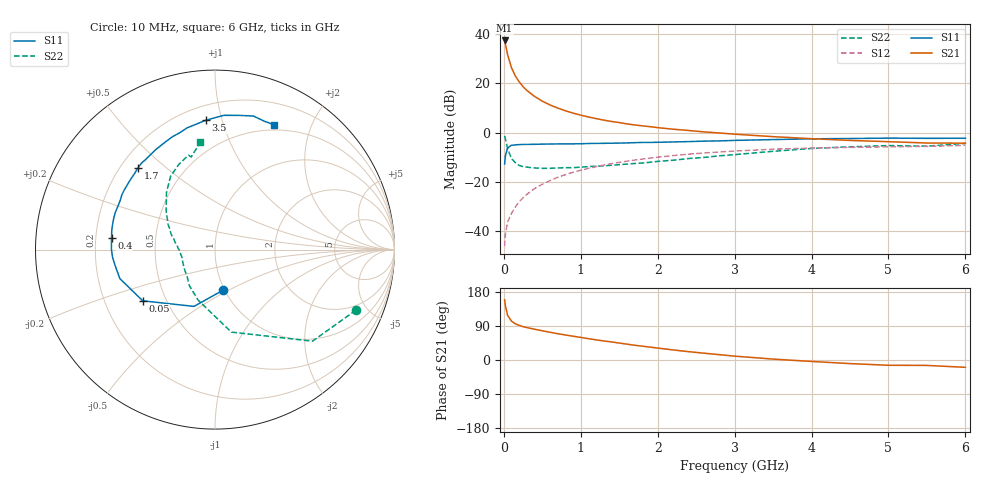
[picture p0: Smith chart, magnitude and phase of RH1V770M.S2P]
! SIEMENS Small Signal Semiconductors
! BFR106
! Si NPN RF Bipolar Junction Transistor in SOT23
! VCE = 1.75 V  IC = 70 mA
! Common Emitter S-Parameters:  August  1996
# GHz  S  MA  R  50
!  f  S11  S21  S12  S22
! GHz  MAG  ANG  MAG  ANG  MAG  ANG  MAG  ANG
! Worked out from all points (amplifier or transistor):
!   36 points, 10 MHz to 6 GHz, reference 50 ohm
!   highest |S21| = 37.4 dB at 10 MHz (marker M1)
!   |S21| within 3 dB of that: start of sweep to 30.49 MHz
!   unconditionally stable (mu >= 1): 180.2 MHz to 2.981 GHz; 4.611 GHz to end of sweep
!   at 250 MHz: K = 1.05, MAG = 21.1 dB, |S12| = -26.4 dB
!   at 1.4 GHz: K = 1.07, MAG = 6.9 dB, |S12| = -12.6 dB
!   at 6 GHz: K = 1.01, MAG = -0.3 dB, |S12| = -5.1 dB
!   S11 on the Smith chart (normalised r, x): 10 MHz: 0.98, -0.47; 50 MHz: 0.37, -0.28; 400 MHz: 0.27, +0.05; 1.7 GHz: 0.27, +0.41; 3.5 GHz: 0.29, +0.89; 6 GHz: 0.44, +1.49
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0.01  0.2316 -79.5  73.8 158.8  0.005 77.5  0.8551 -23.2
0.02  0.3375 -110.3  62.68 142.9  0.0089 66.5  0.7452 -43.2
0.05  0.4936 -144.7  37.23 117.4  0.0155 59.2  0.4686 -78.8
0.1  0.5543 -163.1  20.63 102.4  0.0232 63.7  0.2972 -108.3
0.15  0.5643 -171.4  14.04 95.4  0.0311 66.9  0.2459 -125.7
0.2  0.5723 -175.7  10.67 91.3  0.0398 69.8  0.2161 -135.9
0.25  0.5764 -179.5  8.531 87.9  0.0479 70.8  0.2044 -145.0
0.3  0.5774 178.5  7.14 85.5  0.0564 71.9  0.1996 -150.2
0.4  0.5799 173.6  5.412 81.2  0.0736 72.3  0.1925 -159.0
0.5  0.5848 169.8  4.345 77.1  0.09 71.6  0.1889 -164.8
0.6  0.5878 166.0  3.641 73.2  0.1069 70.9  0.1895 -168.3
0.7  0.5908 162.6  3.149 69.4  0.124 69.6  0.1926 -171.6
0.9  0.5923 156.2  2.485 62.8  0.1575 66.7  0.1952 -178.0
1.1  0.6022 149.5  2.076 56.3  0.1891 63.5  0.2051 178.3
1.3  0.6066 144.2  1.791 50.2  0.2202 59.9  0.2125 173.7
1.7  0.6261 133.1  1.432 38.9  0.2782 53.1  0.2368 165.6
2.2  0.6473 120.8  1.173 26.6  0.3428 44.3  0.2756 155.8
2.8  0.6798 106.8  0.984 14.1  0.4053 34.0  0.339 143.2
3.5  0.7227 94.0  0.829 2.4  0.4617 22.9  0.4185 130.2
4.5  0.7596 79.9  0.695 -9.5  0.5027 8.8  0.5156 113.0
5.5  0.7662 68.8  0.616 -14.3  0.5267 0.4  0.5327 104.4
6  0.7694 64.8  0.611 -19.3  0.5528 -6.3  0.6042 97.7
